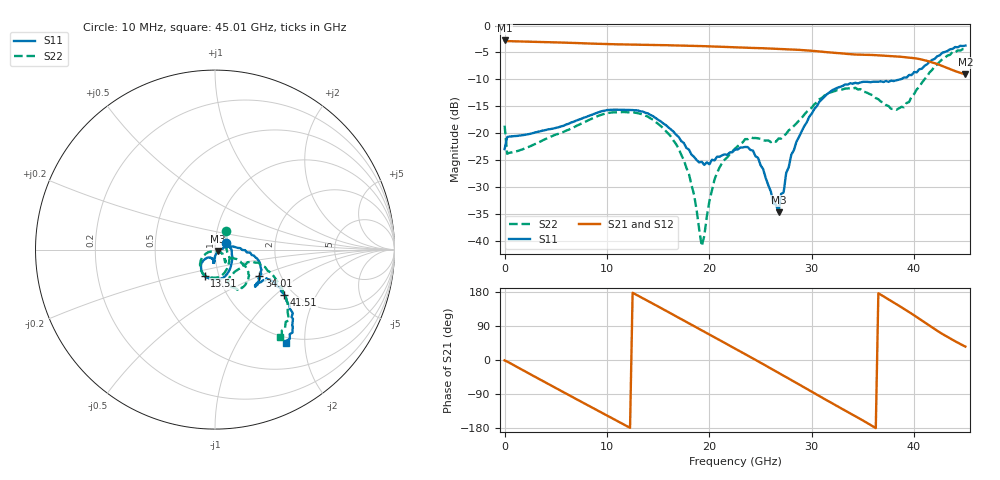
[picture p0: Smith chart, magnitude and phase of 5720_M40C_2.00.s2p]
! Device:  ADRF5720
! Description: 0.5dB LSB GaAs MMIC 6-bit Digital Attenuator
! Frequency:  0.000009 -  40 GHz
! Ports:
!	RF1	= Port 1
!	RF2	= Port 2
! Vdd:  3.3 Volt
! Vss:  -3.3 Volt
! Control:  0/3.3 Volt
! State:  2.00 dB attenuation
! Data:  The device was measured using G-S-G Probes on a matrix board.
!  Data was collected using an calibrated 4 port network analyzer.
!  The reference plane for this measurement is at the launchers.
! Note:  Analog Devices supplies this data as a sample of measured data
!  for this product.  Your particular data for this product may vary.
!  Data was taken at -40 degrees C.
!  Analog Devices reserves the right to change this data at anytime.
# GHZ S DB R 45.0
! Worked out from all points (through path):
!   181 points, 10 MHz to 45.01 GHz, reference 45 ohm
!   highest |S21| = -2.76 dB at 10 MHz (marker M1); lowest = -9.0 dB at 45.01 GHz (marker M2)
!   group delay of S21, straight-line fit = 42 ps
!   lowest |S11| = -34.8 dB at 26.76 GHz (marker M3), VSWR 1.04, Z = 46.5 - j0.708 ohm
!   |S11| at or under -10 dB: start of sweep to 38.66 GHz
!   |S22| runs from -41.0 to -4.4 dB; largest |S21 - S12| = 0.0029
!   S11 on the Smith chart (normalised r, x): 10 MHz: 1.13, +0.08; 13.51 GHz: 0.85, -0.26; 34.01 GHz: 1.56, -0.50; 41.51 GHz: 1.79, -1.14; 45.01 GHz: 0.91, -1.63
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0.01  -22.98 30.2  -2.76 -1.1  -2.78 -1.1  -18.60 59.2
0.26  -20.73 0.2  -2.88 -4.1  -2.89 -4.1  -23.84 1.1
4.26  -19.31 -25.9  -3.09 -63.0  -3.11 -63.0  -20.86 -27.9
7.76  -17.12 -54.4  -3.29 -114.0  -3.30 -114.0  -17.99 -57.9
10.76  -15.64 -82.1  -3.47 -157.3  -3.48 -157.4  -16.13 -87.9
13.51  -16.00 -111.5  -3.58 163.0  -3.59 162.9  -16.52 -117.4
15.26  -17.82 -127.2  -3.62 137.4  -3.64 137.4  -18.67 -135.7
16.76  -20.32 -135.6  -3.69 115.4  -3.70 115.3  -22.07 -149.3
18.01  -23.07 -134.9  -3.74 96.9  -3.76 96.8  -27.60 -159.7
18.51  -24.42 -132.1  -3.77 89.5  -3.78 89.4  -31.46 -154.4
19.26  -25.33 -122.1  -3.81 78.4  -3.82 78.3  -41.04 -108.5
20.51  -25.08 -100.7  -3.89 59.9  -3.91 59.8  -28.62 -25.0
22.76  -23.08 -96.3  -4.05 26.4  -4.07 26.3  -22.46 -44.0
24.76  -24.61 -94.3  -4.18 -3.3  -4.19 -3.5  -20.97 -50.4
26.76  -34.76 -24.6  -4.33 -33.7  -4.35 -33.8  -21.01 -34.8
28.01  -23.99 11.0  -4.43 -52.8  -4.45 -53.0  -19.15 -26.6
30.26  -15.51 -1.1  -4.72 -87.7  -4.74 -87.8  -14.62 -28.7
34.01  -10.81 -30.8  -5.34 -144.6  -5.36 -144.8  -11.74 -54.6
37.76  -10.23 -40.0  -5.67 155.9  -5.69 155.7  -15.49 -60.1
39.01  -9.66 -31.6  -5.86 134.9  -5.88 134.7  -15.20 -31.1
41.51  -6.74 -33.0  -6.70 90.4  -6.72 90.2  -8.71 -25.1
45.01  -3.72 -52.7  -9.03 35.4  -9.06 35.2  -4.36 -53.3
